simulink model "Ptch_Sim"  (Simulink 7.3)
settings: Solver=ode45  StartTime=0.0  StopTime=20  RelTol=1e-3
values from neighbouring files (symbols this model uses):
  Api = [    [pitch_115.m]    (also in pitch_195.m; pitch_290.m; pitch_395.m; pitch_455.m)
  Bpi = [    [pitch_115.m]    (also in pitch_195.m; pitch_290.m; pitch_395.m; pitch_455.m)
  Cpi = [    [pitch_115.m]    (also in pitch_195.m; pitch_290.m; pitch_395.m; pitch_455.m)
  Dpi = [    [pitch_115.m]    (also in pitch_195.m; pitch_290.m; pitch_395.m; pitch_455.m)
undefined symbols (not defined in the file or in its folder): Kq

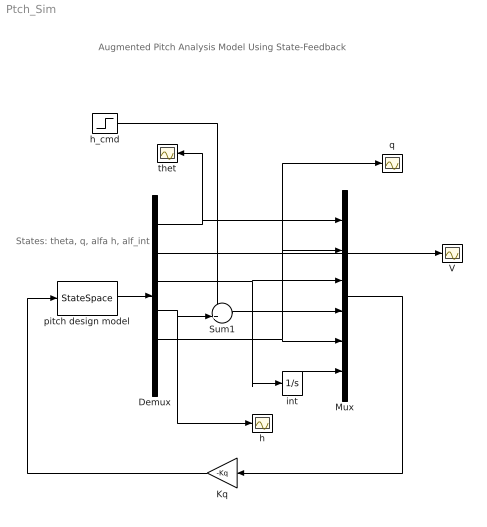
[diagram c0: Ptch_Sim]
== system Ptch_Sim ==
  note: Augmented Pitch Analysis Model Using State-Feedback
  note: States: theta, q, alfa h, alf_int
  Demux : Demux  Outputs=6
  Kq : Gain  Gain=-Kq  Multiplication=Matrix(K*u)  ParameterDataType=fixdt(1, 16)  ParameterScaling=2^0  OutDataType=fixdt(1, 16)  OutScaling=2^0
  Mux : Mux  Inputs=6
  Sum1 : Sum  Inputs=-+|  OutDataType=fixdt(1, 16)  OutScaling=2^0
  V : Scope
  h : Scope
  h_cmd : Step  Time=0  SampleTime=0
  int : Integrator
  pitch design model : StateSpace  A=Api  B=Bpi  C=Cpi  D=Dpi
  q : Scope
  thet : Scope
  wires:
  Kq/1 -> pitch design model/1
  Demux/4 -> Sum1/2, h/1
  Sum1/1 -> Mux/4
  h_cmd/1 -> Sum1/1
  pitch design model/1 -> Demux/1
  Demux/1 -> thet/1, Mux/1
  Demux/2 -> Mux/2, q/1
  Demux/3 -> Mux/3, int/1
  Demux/5 -> Mux/5, V/1
  Mux/1 -> Kq/1
  int/1 -> Mux/6
